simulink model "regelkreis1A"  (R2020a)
settings: Solver=ode45  StartTime=0.0  StopTime=10  MaxStep=0.01  RelTol=1e-3  EnableMultiTasking=on

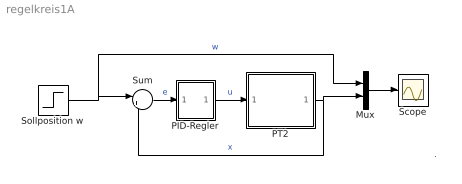
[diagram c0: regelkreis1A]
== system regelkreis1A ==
  note: .
  Mux : Mux  Inputs=2
  PID-Regler : Subsystem  mask(PID-Regler){Kp=10, Ki=20, Kd=5}
      mask prompts: Kp "Proportional"; Ki "Integral"; Kd "Differentiell"
      mask help: Regler mit Proportional-, Integral- und Ableitungsanteil.
  PT2 : Subsystem  mask(PT2){D=0.2, om0=3, b0=1.0}
      mask prompts: D "Daempfungsgrad"; om0 "Eigenfrequenz"; b0 "Staerke"
      mask help: schwingfaehige Regelstrecke mit Daempfung D Eigenfrequenz om0 Starke b0
  Scope : Scope
  Sollposition w : Step  SampleTime=0
  Sum : Sum  Inputs=|+-  SaturateOnIntegerOverflow=on
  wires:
  PID-Regler/1(u) -> PT2/1(u)  "u"
  PT2/1(x) -> Sum/2, Mux/2  "x"
  Sollposition w/1 -> Sum/1, Mux/1  "w"
  Mux/1 -> Scope/1
  Sum/1 -> PID-Regler/1(e)  "e"

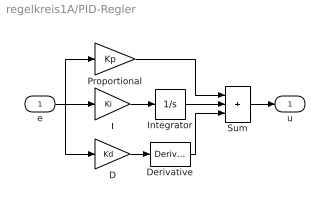
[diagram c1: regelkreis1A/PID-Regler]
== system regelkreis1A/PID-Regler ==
  e : Inport
  D : Gain  Gain=Kd  SaturateOnIntegerOverflow=on
  Derivative : Derivative
  I : Gain  Gain=Ki  SaturateOnIntegerOverflow=on
  Integrator : Integrator
  Proportional : Gain  Gain=Kp  SaturateOnIntegerOverflow=on
  Sum : Sum  Inputs=+++  InputSameDT=on  SaturateOnIntegerOverflow=on
  u : Outport  InitialOutput=0
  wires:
  I/1 -> Integrator/1
  Proportional/1 -> Sum/1
  Integrator/1 -> Sum/2
  Derivative/1 -> Sum/3
  e/1 -> I/1, Proportional/1, D/1
  Sum/1 -> u/1
  D/1 -> Derivative/1

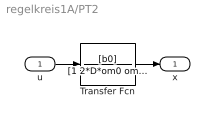
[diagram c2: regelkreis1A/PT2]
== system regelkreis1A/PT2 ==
  u : Inport
  Transfer Fcn : TransferFcn  Numerator=[b0]  Denominator=[1 2*D*om0 om0*om0]
  x : Outport
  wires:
  Transfer Fcn/1 -> x/1
  u/1 -> Transfer Fcn/1
